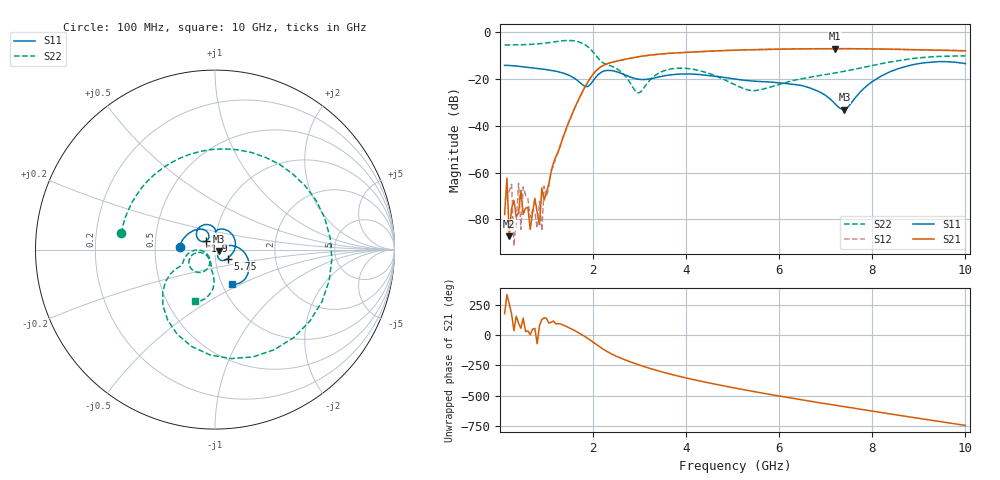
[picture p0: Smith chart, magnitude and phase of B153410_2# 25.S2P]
!  2-Port S-parameters saved by WinCal
! VAR MeasName=S-Parameters (CALIBRATED_DATA) read from VNA (N5245A)
! VAR MeasDate=2016-12-23 10:00:37
! VAR NAME=B153410_2# 25
! VAR FILENAME=B153410_2# 25.S2P
! VAR DATE=2016-12-23 10:00:38
! VAR PHYS_PORTS=1,2
# Hz S DB R 50
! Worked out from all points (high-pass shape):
!   199 points, 100 MHz to 10 GHz, reference 50 ohm
!   highest |S21| = -7.06 dB at 7.2 GHz (marker M1); lowest = -87.1 dB at 200 MHz (marker M2)
!   |S21| within 3 dB of the highest: 3.127 GHz to end of sweep
!   lowest |S11| = -33.1 dB at 7.4 GHz (marker M3), VSWR 1.05, Z = 52.1 - j0.832 ohm
!   |S11| at or under -10 dB: start of sweep to end of sweep
!   |S22| runs from -25.9 to -3.6 dB; largest |S21 - S12| = 0.0035
!   S11 on the Smith chart (normalised r, x): 100 MHz: 0.67, +0.02; 1.9 GHz: 0.90, +0.08; 5.75 GHz: 1.15, -0.12; 10 GHz: 1.11, -0.45
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1e8  -14.19 175.4  -77.91 178.2  -71.45 77.0  -5.52 170.2
1.5e8  -14.20 172.8  -62.33 -23.5  -70.63 -34.5  -5.51 165.3
2e8  -14.24 170.5  -87.14 -99.8  -67.88 -178.4  -5.50 160.4
3.5e8  -14.49 163.2  -78.84 157.3  -80.24 145.9  -5.48 145.0
4e8  -14.60 161.2  -77.07 98.2  -64.56 52.4  -5.44 139.8
4.5e8  -14.69 159.0  -67.58 58.1  -84.27 165.0  -5.42 134.3
5e8  -14.80 156.9  -77.81 141.4  -66.05 87.7  -5.39 128.8
6.5e8  -15.15 150.8  -84.29 3.2  -79.14 44.6  -5.26 111.1
8.5e8  -15.62 143.2  -82.20 80.7  -72.15 67.1  -4.98 84.4
9e8  -15.76 141.2  -66.58 129.3  -84.83 165.8  -4.87 77.1
1.35e9  -17.46 122.4  -45.17 85.0  -45.43 84.5  -3.70 -4.5
1.75e9  -22.08 115.4  -26.41 6.7  -26.36 6.8  -4.62 -92.7
1.9e9  -23.09 138.4  -20.93 -30.2  -20.96 -30.2  -6.50 -123.8
2.95e9  -20.05 88.0  -10.63 118.8  -10.63 118.7  -25.89 -151.1
3.4e9  -19.18 83.2  -9.47 64.6  -9.47 64.6  -17.66 -115.2
5.05e9  -20.06 -12.2  -7.72 -78.2  -7.73 -78.0  -22.51 -165.8
5.75e9  -21.20 -35.2  -7.38 -127.4  -7.39 -127.1  -23.79 -118.3
6.7e9  -24.16 -64.2  -7.11 170.8  -7.11 170.9  -19.11 -99.8
7.2e9  -30.63 -58.8  -7.06 139.5  -7.08 139.6  -17.47 -95.4
7.4e9  -33.07 -21.0  -7.08 127.3  -7.08 127.3  -16.73 -93.7
8.35e9  -17.22 2.6  -7.29 69.5  -7.29 69.8  -12.85 -93.9
1e10  -13.45 -63.7  -7.98 -27.7  -7.98 -27.3  -10.17 -111.5
